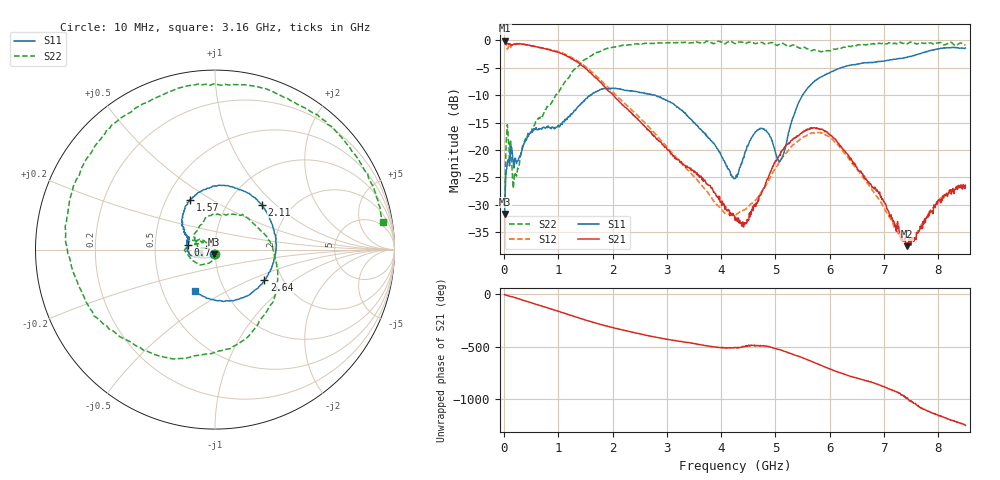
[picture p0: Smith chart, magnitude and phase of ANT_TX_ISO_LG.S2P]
!Agilent Technologies,E5071C,MY46523237,B.13.01
!Date: Tue Sep 12 16:56:35 2023
!Data & Calibration Information:
!Freq	S11:SOLT2(ON)	S21:SOLT2(ON)	S12:SOLT2(ON)	S22:SOLT2(ON)
!PortZ  Port1:50+j0  Port2:50+j0
!Above PortZ is port z conversion or system Z0 setting when saving the data.
!When reading, reference impedance value at option line is always used.
# Hz S dB R 50
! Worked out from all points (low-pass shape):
!   850 points, 10 MHz to 8.5 GHz, reference 50 ohm
!   highest |S21| = -0.13 dB at 10 MHz (marker M1); lowest = -37.5 dB at 7.42 GHz (marker M2)
!   |S21| within 3 dB of the highest: start of sweep to 1.199 GHz
!   lowest |S11| = -31.6 dB at 10 MHz (marker M3), VSWR 1.05, Z = 49.3 - j2.52 ohm
!   |S11| at or under -10 dB: start of sweep to 1.596 GHz; 2.753198 GHz to 2.764492 GHz (11.29 MHz wide, 0.409 % of centre); 2.776 GHz to 5.498 GHz (2.723 GHz wide, 65.8 % of centre)
!   |S22| runs from -31.9 to -0.1 dB; largest |S21 - S12| = 0.11
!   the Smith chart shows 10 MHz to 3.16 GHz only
!   S11 on the Smith chart (normalised r, x): 10 MHz: 0.99, -0.05; 700 MHz: 0.73, +0.04; 1.57 GHz: 0.66, +0.41; 2.11 GHz: 1.42, +0.82; 2.64 GHz: 1.62, -0.61; 3.16 GHz: 0.73, -0.35
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1e7  -31.64 -103.2  -0.13 -2.5  -0.06 -3.1  -31.95 -90.5
8e7  -21.78 -155.5  -0.67 -14.4  -1.17 -10.6  -18.48 155.0
2e8  -21.48 -163.9  -0.75 -32.3  -0.70 -30.6  -24.08 170.7
7e8  -16.17 170.0  -1.43 -113.2  -1.40 -111.9  -13.88 76.7
1.06e9  -15.17 155.0  -2.45 -172.1  -2.27 -170.9  -8.52 -21.2
1.43e9  -11.40 131.6  -4.61 125.9  -4.30 127.5  -4.02 -105.5
1.57e9  -10.16 116.2  -5.82 103.6  -5.38 104.7  -3.14 -132.1
2.11e9  -8.84 44.0  -11.00 28.8  -10.50 28.4  -1.15 141.7
2.64e9  -9.81 -31.5  -16.21 -32.6  -15.50 -36.4  -0.53 73.0
2.84e9  -10.27 -63.6  -18.24 -54.1  -17.69 -58.8  -0.56 48.3
3.16e9  -11.93 -115.8  -21.62 -81.9  -21.24 -90.6  -0.47 9.3
3.74e9  -17.48 169.2  -26.20 -130.9  -27.57 -135.5  -0.21 -59.2
4.26e9  -25.14 36.0  -32.84 -149.3  -31.80 -136.8  -0.62 -117.0
4.95e9  -18.76 -139.8  -22.95 -150.3  -24.11 -158.6  -0.43 164.0
5.35e9  -13.37 -94.1  -17.74 141.9  -18.88 141.7  -0.92 103.3
5.67e9  -7.95 -130.1  -16.07 79.0  -16.90 80.8  -1.93 29.2
6.1e9  -5.47 -174.6  -17.97 -12.5  -18.61 -9.4  -1.66 -98.5
6.5e9  -4.40 146.4  -23.16 -78.9  -23.49 -78.4  -0.93 178.1
7.09e9  -3.64 89.1  -31.29 177.4  -32.01 -176.7  -0.50 103.6
7.42e9  -3.14 55.3  -37.51 89.6  -36.98 87.3  -0.70 70.1
8.01e9  -1.58 -19.2  -29.07 -78.0  -29.11 -75.7  -0.48 13.0
8.5e9  -1.44 -103.0  -26.40 -171.4  -26.46 -168.1  -0.92 -36.5
